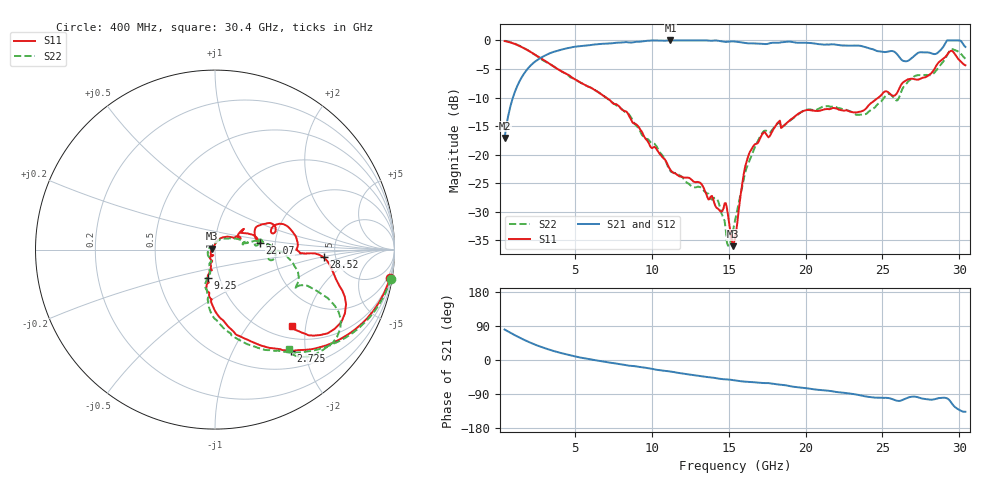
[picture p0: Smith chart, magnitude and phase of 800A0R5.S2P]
!  American Technical Ceramics  Date:  9/12/2007
!  One Norden Lane
!  Huntington Station,  NY.  11746-2102
!  Tel:  (631) 622-4700  Fax:  (631) 622-4748
!  Part Number  800A0R5  Mounting Orientation: Vertical
!  Description: Ultra Low ESR Microwave capacitors
!  Application: Coupling, Bypass, Tuning, DC Block
!  Filters, Matching
# GHZ S DB R 50
! Freq  |S11|  S11 Ph  |S21|  S21 Ph  |S12|  S12 Ph  |S22|  S22 Ph
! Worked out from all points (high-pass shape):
!   401 points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, 400 MHz to 30.4 GHz, reference 50 ohm
!   highest |S21| = -0.01 dB at 11.2 GHz (marker M1); lowest = -17.1 dB at 400 MHz (marker M2)
!   |S21| within 3 dB of the highest: 2.773 GHz to 26.13 GHz (23.36 GHz wide, 162 % of centre); 26.95 GHz to end of sweep
!   lowest |S11| = -36.0 dB at 15.25 GHz (marker M3), VSWR 1.03, Z = 48.5 + j0.426 ohm
!   |S11| at or under -10 dB: 7.005 GHz to 24.74 GHz (17.74 GHz wide, 112 % of centre)
!   |S22| runs from -35.9 to -0.1 dB; largest |S21 - S12| = 0.0025
!   S11 on the Smith chart (normalised r, x): 400 MHz: 1, -12; 2.725 GHz: 0.78, -1.73; 9.25 GHz: 0.88, -0.29; 22.07 GHz: 1.66, +0.13; 28.52 GHz: 4.01, -0.55; 30.4 GHz: 1.25, -1.68
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0.4  -0.12 -9.4  -17.09 80.4  -17.07 80.3  -0.07 -9.3
1.3  -0.89 -28.9  -7.53 60.6  -7.53 60.5  -0.84 -29.4
2.725  -3.06 -53.2  -3.08 35.2  -3.08 35.1  -3.17 -55.2
5.425  -7.50 -81.4  -0.98 5.7  -0.98 5.7  -7.50 -85.7
9.25  -15.67 -104.1  -0.21 -18.6  -0.21 -18.6  -16.07 -106.5
10.45  -19.69 -103.2  -0.04 -26.7  -0.04 -26.7  -19.29 -107.2
11.2  -22.65 -106.0  -0.01 -30.4  -0.01 -30.5  -22.87 -108.3
14.2  -29.30 -116.8  -0.02 -48.3  -0.03 -48.4  -27.70 -174.2
14.8  -28.49 -123.6  -0.27 -51.0  -0.27 -51.0  -33.17 139.0
15.25  -36.01 163.9  -0.18 -53.0  -0.18 -53.1  -33.95 130.8
15.4  -34.63 121.1  -0.20 -54.1  -0.20 -54.1  -31.57 112.7
16  -22.91 63.0  -0.44 -57.0  -0.45 -57.0  -23.88 62.7
16.525  -18.79 37.1  -0.53 -58.4  -0.52 -58.5  -19.78 37.5
20.425  -12.27 9.9  -0.50 -76.7  -0.50 -76.8  -12.15 9.1
22.075  -11.99 8.3  -0.79 -84.8  -0.78 -84.8  -11.80 8.3
23.8  -12.21 25.6  -1.10 -95.3  -1.09 -95.5  -12.97 8.9
25.45  -9.25 15.8  -1.91 -100.9  -1.91 -100.9  -9.40 -5.9
26.425  -7.18 14.4  -3.62 -103.3  -3.64 -103.4  -7.95 -5.2
28.525  -4.34 -4.1  -2.31 -101.9  -2.31 -102.0  -5.18 -21.4
29.275  -2.28 -19.9  -0.01 -102.9  -0.01 -102.8  -2.27 -26.7
29.875  -3.01 -42.5  -0.01 -128.7  -0.01 -128.7  -1.86 -46.6
30.4  -4.36 -44.7  -1.14 -136.6  -1.14 -136.6  -3.20 -53.5
